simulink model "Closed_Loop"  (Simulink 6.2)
settings: Solver=ode23s  StartTime=0.0  StopTime=60  FixedStep=0.04  RelTol=1e-3
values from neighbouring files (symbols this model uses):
  r2d = 180/pi    (= 57.2957795131)    [run.m]    (also in Pl.m; pl.m; start.m)
undefined symbols (not defined in the file or in its folder): Ac, As, At, Av, Bc, Bs, Bt, Bv, Cc, Cs, Ct, Cv, Dc, Ds, Dt, Dv

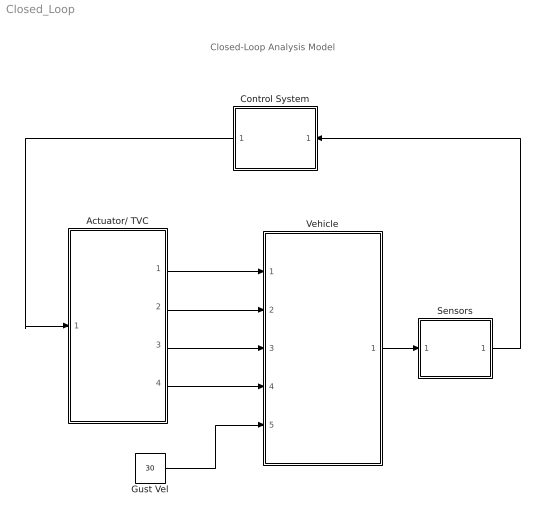
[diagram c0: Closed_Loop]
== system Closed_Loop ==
  note: Closed-Loop Analysis Model
  Actuator/ TVC : Subsystem
  Control System : Subsystem  Orientation=left
  Gust Vel : Constant  Value=30
  Sensors : Subsystem
  Vehicle : Subsystem
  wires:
  Vehicle/1(meas) -> Sensors/1(meas)
  Actuator/ TVC/1(DY) -> Vehicle/1(DY)
  Actuator/ TVC/2(DY-dd) -> Vehicle/2(DY_dd)
  Actuator/ TVC/3(DZ) -> Vehicle/3(DZ)
  Actuator/ TVC/4(DZ-dd) -> Vehicle/4(DZ_dd)
  Sensors/1(sens) -> Control System/1(sens)
  Control System/1(TVC) -> Actuator/ TVC/1(TVC)
  Gust Vel/1 -> Vehicle/5(Vgust)

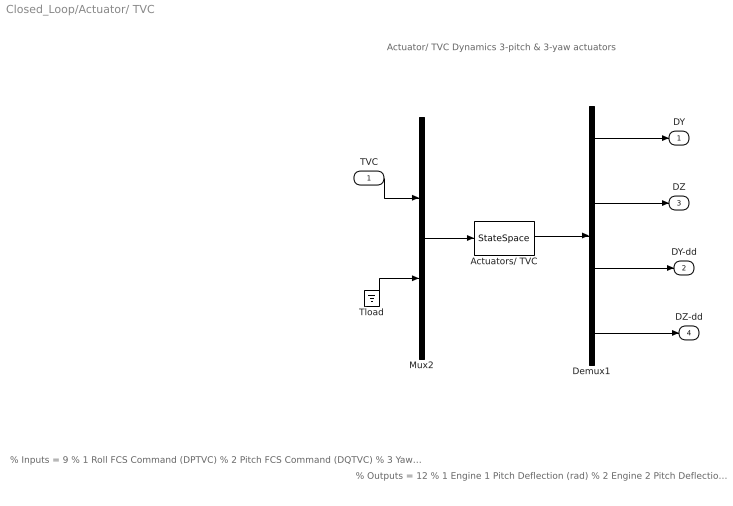
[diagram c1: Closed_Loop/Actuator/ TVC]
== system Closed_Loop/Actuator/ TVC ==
  note: % Outputs = 12 % 1 Engine 1 Pitch Deflection (rad) % 2 Engine 2 Pitch Deflection (rad) % 3 Engine 3 Pitch Deflection (rad) % 4 Engine 1 Yaw Deflection (rad) % 5 Engine 2 Yaw Deflection (rad) % 6 Engine 3 Yaw Deflection (rad) % 7 Engine 1 Pitch Accelerat (rad/sec^2) % 8 Engine 2 Pitch Accelerat (rad/sec^2) % 9 Engine 3 Pitch Accelerat (rad/sec^2) % 10 Engine 1 Yaw Accelerat (rad/sec^2) % 11 Engine 2 Yaw Accelerat (rad/sec^2) % 12 Engine 3 Yaw Accelerat (rad/sec^2)
  note: % Inputs = 9 % 1 Roll FCS Command (DPTVC) % 2 Pitch FCS Command (DQTVC) % 3 Yaw FCS Command (DRTVC) % 4 Engine 1 Pitch Load-Torque TLY1 % 5 Engine 2 Pitch Load-Torque TLY2 % 6 Engine 3 Pitch Load-Torque TLY3 % 7 Engine 1 Yaw Load-Torque TLZ1 % 8 Engine 2 Yaw Load-Torque TLZ2 % 9 Engine 3 Yaw Load-Torque TLZ3
  note: Actuator/ TVC Dynamics 3-pitch & 3-yaw actuators
  TVC : Inport  Port=1  LatchInput=off
  Actuators/ TVC : StateSpace  A=At  B=Bt  C=Ct  D=Dt
  Demux1 : Demux  Outputs=[3, 3, 3, 3]
  Mux2 : Mux  Inputs="[3,  6]"
  Tload : Ground
  DY : Outport
  DY-dd : Outport  Port=2
  DZ : Outport  Port=3
  DZ-dd : Outport  Port=4
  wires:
  Demux1/3 -> DY-dd/1
  Demux1/4 -> DZ-dd/1
  Demux1/2 -> DZ/1
  Demux1/1 -> DY/1
  TVC/1 -> Mux2/1
  Tload/1 -> Mux2/2
  Actuators/ TVC/1 -> Demux1/1
  Mux2/1 -> Actuators/ TVC/1

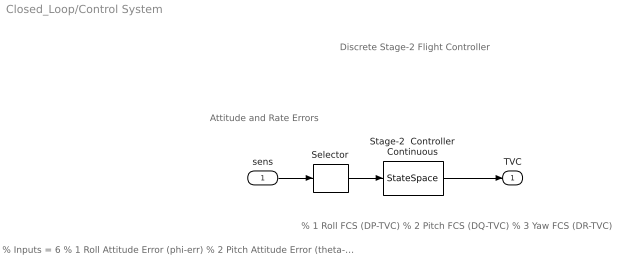
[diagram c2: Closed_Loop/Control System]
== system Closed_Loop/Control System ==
  note: Discrete Stage-2 Flight Controller
  note: Attitude and Rate Errors
  note: % Inputs = 6 % 1 Roll Attitude Error (phi-err) % 2 Pitch Attitude Error (theta-err) % 3 Yaw Attitude Error (psi-err) % 4 Roll Rate Error (p-err) % 5 Pitch Rate Error (q-err) % 6 Yaw Rate Error (r-err)
  note: % 1 Roll FCS (DP-TVC) % 2 Pitch FCS (DQ-TVC) % 3 Yaw FCS (DR-TVC)
  sens : Inport  Port=1  LatchInput=off
  Selector : Selector  Elements=[1 3 5 2 4 6]  InputPortWidth=6
  Stage-2  Controller Continuous : StateSpace  A=Ac  B=Bc  C=Cc  D=Dc
  TVC : Outport
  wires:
  sens/1 -> Selector/1
  Stage-2  Controller Continuous/1 -> TVC/1
  Selector/1 -> Stage-2  Controller Continuous/1

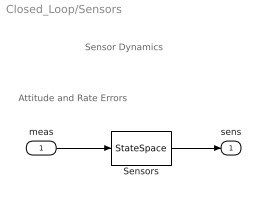
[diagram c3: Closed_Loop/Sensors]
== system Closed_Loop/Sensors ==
  note: Attitude and Rate Errors
  note: Sensor Dynamics
  meas : Inport  Port=1  LatchInput=off
  Sensors : StateSpace  A=As  B=Bs  C=Cs  D=Ds
  sens : Outport
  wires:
  Sensors/1 -> sens/1
  meas/1 -> Sensors/1

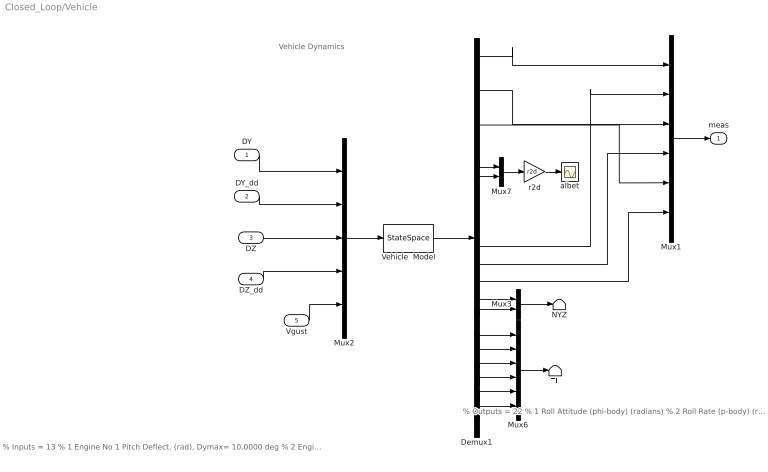
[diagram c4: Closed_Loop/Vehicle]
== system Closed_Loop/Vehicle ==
  note: % Outputs = 22 % 1 Roll Attitude (phi-body) (radians) % 2 Roll Rate (p-body) (rad/sec) % 3 Pitch Attitude (thet-bdy) (radians) % 4 Pitch Rate (q-body) (rad/sec) % 5 Yaw Attitude (psi-body) (radians) % 6 Yaw Rate (r-body) (rad/sec) % 7 Angle of attack, alfa, (radians) % 8 Angle of sideslip, beta, (radian) % 9 Change in Altitude, delta-h, (feet) % 10 Forward Acceleration (V-dot) (ft/sec) % 11 Cross Range Velocity (Vcr) (ft/sec) % 12 Rate-Gyro # 1, Roll Rate (Body) (rad/sec) % 13 Rate-Gyro # 2, Pitch Rate (Body) (rad/sec) % 14 Rate-Gyro # 3, Yaw Rate (Body) (rad/sec) % 15 Accelerom # 1, (along Z), (ft/sec^2) Translat. Acceler % 16 Accelerom # 2, (along Y), (ft/sec^2) Translat. Acceler % 17 Ptch Load-Torque Tly for Engine: 1,(ft-lb) % 18 Ptch Load-Torque Tly for Engine: 2,(ft-lb) % 19 Ptch Load-Torque Tly for Engine: 3,(ft-lb) % 20 Yaw Load-Torque Tlz for Engine: 1,(ft-lb) % 21 Yaw Load-Torque Tlz for Engine: 2,(ft-lb) % 22 Yaw Load-Torque Tlz for Engine: 3,(ft-lb)
  note: % Inputs = 13 % 1 Engine No 1 Pitch Deflect. (rad), Dymax= 10.0000 deg % 2 Engine No 2 Pitch Deflect. (rad), Dymax= 10.0000 deg % 3 Engine No 3 Pitch Deflect. (rad), Dymax= 10.0000 deg % 4 Engine No 1 Pitch Acceleration (rad/sec^2) % 5 Engine No 2 Pitch Acceleration (rad/sec^2) % 6 Engine No 3 Pitch Acceleration (rad/sec^2) % 7 Engine No 1 Yaw Deflect. (rad), Dzmax= 10.0000 deg % 8 Engine No 2 Yaw Deflect. (rad), Dzmax= 10.0000 deg % 9 Engine No 3 Yaw Deflect. (rad), Dzmax= 10.0000 deg % 10 Engine No 1 Yaw Acceleration (rad/sec^2) % 11 Engine No 2 Yaw Acceleration (rad/sec^2) % 12 Engine No 3 Yaw Acceleration (rad/sec^2) % 13 Wind Gust Azim, Elev Angles=( 45.0 90.0) (deg)
  note: Vehicle Dynamics
  DY : Inport  Port=1  LatchInput=off
  DY_dd : Inport  Port=2  LatchInput=off
  DZ : Inport  Port=3  LatchInput=off
  DZ_dd : Inport  Port=4  LatchInput=off
  Vgust : Inport  Port=5  LatchInput=off
  Demux1 : Demux  Outputs=22
  Mux1 : Mux  Inputs=6
  Mux2 : Mux  Inputs=[3, 3, 3, 3, 1]
  Mux3 : Mux  Inputs=2
  Mux6 : Mux  Inputs=6
  Mux7 : Mux  Inputs=2
  NYZ : Terminator
  TL : Terminator
  Vehicle  Model : StateSpace  A=Av  B=Bv  C=Cv  D=Dv
  albet : Scope
  r2d : Gain  Gain=r2d
  meas : Outport
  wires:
  Mux1/1 -> meas/1
  Demux1/5 -> Mux1/5
  Demux1/3 -> Mux1/3
  Demux1/1 -> Mux1/1
  DZ_dd/1 -> Mux2/4
  Vgust/1 -> Mux2/5
  DZ/1 -> Mux2/3
  DY_dd/1 -> Mux2/2
  DY/1 -> Mux2/1
  Demux1/8 -> Mux7/2
  Demux1/7 -> Mux7/1
  Demux1/12 -> Mux1/2
  Demux1/13 -> Mux1/4
  Demux1/14 -> Mux1/6
  Mux6/1 -> TL/1
  Demux1/17 -> Mux6/1
  Demux1/18 -> Mux6/2
  Demux1/19 -> Mux6/3
  Demux1/20 -> Mux6/4
  Demux1/21 -> Mux6/5
  Demux1/22 -> Mux6/6
  Mux3/1 -> NYZ/1
  Demux1/16 -> Mux3/2
  Demux1/15 -> Mux3/1
  Vehicle  Model/1 -> Demux1/1
  Mux2/1 -> Vehicle  Model/1
  r2d/1 -> albet/1
  Mux7/1 -> r2d/1
